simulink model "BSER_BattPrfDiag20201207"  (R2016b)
settings: Solver=FixedStepDiscrete  StartTime=0.0  StopTime=10.0  FixedStep=0.02  RelTol=1e-3  EnableMultiTasking=on
undefined symbols (not defined in the file or in its folder): bin2dec, BSER_cntBattOCMinDiag_C, BSER_cntBattPrfDiag_CW, BSER_cntChrgOCNpl_C, BSER_cntDisChOCNpl_C, BSER_cntPwrConvertConst_C, BSER_iChrgCurrErr_C, BSER_iChrgCurrOk_C, BSER_iDisChCurrErr_C, BSER_iDisChCurrOk_C, BSER_iLonChrgCurrErr_C, BSER_iLonChrgCurrOk_C, BSER_iLonDisChCurrErr_C, BSER_iLonDisChCurrOk_C, BSER_iShrtChrgCurrErr_C, BSER_iShrtChrgCurrOk_C, BSER_iShrtDisChCurrErr_C, BSER_iShrtDisChCurrOk_C, BSER_iSumLonChrgCurrReq_C, BSER_iSumLonDisChCurrReq_C, BSER_iSumShrtChrgCurrReq_C, BSER_iSumShrtDisChCurrReq_C, BSER_rLonChrgCurrHeal_C, BSER_rLonChrgCurrHi_C, BSER_rLonDisChCurrHeal_C, BSER_rLonDisChCurrHi_C, BSER_rShrtChrgCurrHeal_C, BSER_rShrtChrgCurrHi_C, BSER_rShrtDisChCurrHeal_C, BSER_rShrtDisChCurrHi_C, BSER_tiChrgCurrErr_C, BSER_tiChrgCurrOk_C, BSER_tiCurrConstPer_C, BSER_tiCurrPeakPer_C, BSER_tiDisChCurrErr_C, BSER_tiDisChCurrOk_C, BSER_uBattVoltConst_C
libraries: simulink x68
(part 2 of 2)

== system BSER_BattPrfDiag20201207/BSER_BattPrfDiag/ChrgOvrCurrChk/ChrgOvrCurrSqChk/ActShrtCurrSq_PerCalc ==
  BSPR_iCurr : Inport
  BSER_tiCurrConstPer_C : Inport  Port=2
  CurrProc : Stateflow chart  TreatAsAtomicUnit=on
  Sum of Elements : Sum  Inputs=+
  Terminator : Terminator
  Terminator1 : Terminator
  BSER_iCurrPerAcm : Outport
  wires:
  CurrProc/2(Index_s) -> Terminator/1
  CurrProc/3(i) -> Terminator1/1
  CurrProc/1(BSER_iCurrSqAvrgS_A) -> Sum of Elements/1
  BSPR_iCurr/1 -> CurrProc/1(BSPR_iCurr)
  Sum of Elements/1 -> BSER_iCurrPerAcm/1
  BSER_tiCurrConstPer_C/1 -> CurrProc/2(BSER_tiCurrCalcPer_C)

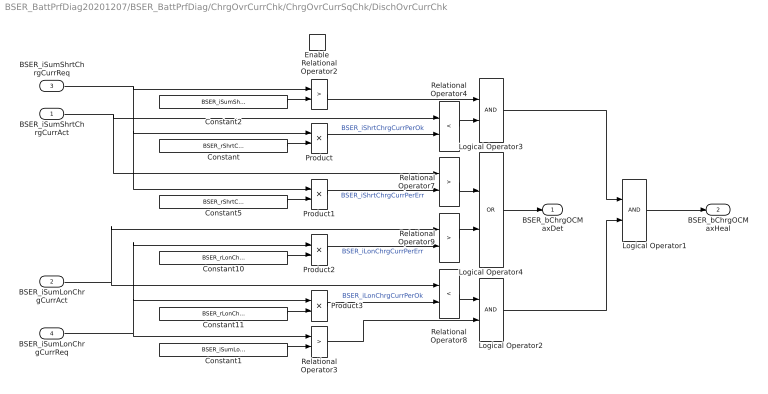
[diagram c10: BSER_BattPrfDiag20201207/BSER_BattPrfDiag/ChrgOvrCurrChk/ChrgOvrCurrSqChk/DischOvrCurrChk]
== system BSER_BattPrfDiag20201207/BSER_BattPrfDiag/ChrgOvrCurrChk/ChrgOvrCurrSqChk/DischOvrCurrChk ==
  BSER_iSumShrtChrgCurrAct : Inport
  BSER_iSumLonChrgCurrAct : Inport  Port=2
  BSER_iSumShrtChrgCurrReq : Inport  Port=3
  BSER_iSumLonChrgCurrReq : Inport  Port=4
  Enable : EnablePort
  Constant : Constant  Value=BSER_rShrtChrgCurrHeal_C
  Constant1 : Constant  Value=BSER_iSumLonChrgCurrReq_C
  Constant10 : Constant  Value=BSER_rLonChrgCurrHi_C
  Constant11 : Constant  Value=BSER_rLonChrgCurrHeal_C
  Constant2 : Constant  Value=BSER_iSumShrtChrgCurrReq_C
  Constant5 : Constant  Value=BSER_rShrtChrgCurrHi_C
  Logical Operator1 : Logic  AllPortsSameDT=off  OutDataTypeStr=boolean
  Logical Operator2 : Logic  AllPortsSameDT=off  OutDataTypeStr=boolean
  Logical Operator3 : Logic  AllPortsSameDT=off  OutDataTypeStr=boolean
  Logical Operator4 : Logic  Operator=OR  AllPortsSameDT=off  OutDataTypeStr=boolean
  Product{,1..3} (4 alike) : Product
  Relational Operator{2..3,7,9} (4 alike) : RelationalOperator  Operator=>  OutDataTypeStr=boolean  RndMeth=Simplest
  Relational Operator4 : RelationalOperator  Operator=<  OutDataTypeStr=boolean  RndMeth=Simplest
  Relational Operator8 : RelationalOperator  Operator=<  OutDataTypeStr=boolean  RndMeth=Simplest
  BSER_bChrgOCMaxDet : Outport
  BSER_bChrgOCMaxHeal : Outport  Port=2
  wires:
  Logical Operator1/1 -> BSER_bChrgOCMaxHeal/1
  Logical Operator4/1 -> BSER_bChrgOCMaxDet/1
  Logical Operator2/1 -> Logical Operator1/2
  Logical Operator3/1 -> Logical Operator1/1
  Relational Operator8/1 -> Logical Operator2/1
  Relational Operator3/1 -> Logical Operator2/2
  Relational Operator2/1 -> Logical Operator3/1
  Constant1/1 -> Relational Operator3/2
  Relational Operator4/1 -> Logical Operator3/2
  Relational Operator9/1 -> Logical Operator4/2
  Relational Operator7/1 -> Logical Operator4/1
  BSER_iSumLonChrgCurrAct/1 -> Relational Operator9/1, Relational Operator8/1
  BSER_iSumLonChrgCurrReq/1 -> Product3/1, Product2/1, Relational Operator3/1
  BSER_iSumShrtChrgCurrAct/1 -> Relational Operator7/1, Relational Operator4/1
  BSER_iSumShrtChrgCurrReq/1 -> Product1/1, Product/1, Relational Operator2/1
  Constant/1 -> Product/2
  Product/1 -> Relational Operator4/2  "BSER_iShrtChrgCurrPerOk"
  Product1/1 -> Relational Operator7/2  "BSER_iShrtChrgCurrPerErr"
  Constant5/1 -> Product1/2
  Constant2/1 -> Relational Operator2/2
  Constant10/1 -> Product2/2
  Product2/1 -> Relational Operator9/2  "BSER_iLonChrgCurrPerErr"
  Product3/1 -> Relational Operator8/2  "BSER_iLonChrgCurrPerOk"
  Constant11/1 -> Product3/2

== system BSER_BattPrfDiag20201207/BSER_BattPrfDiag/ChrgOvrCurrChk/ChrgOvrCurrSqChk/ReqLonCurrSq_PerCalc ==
  BSPR_iCurr : Inport
  BSER_tiCurrConstPer_C : Inport  Port=2
  CurrProc1 : Stateflow chart  TreatAsAtomicUnit=on
  Sum of Elements : Sum  Inputs=+
  Terminator : Terminator
  Terminator1 : Terminator
  BSER_iCurrPerAcm : Outport
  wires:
  BSER_tiCurrConstPer_C/1 -> CurrProc1/2(BSER_tiCurrCalcPer_C)
  Sum of Elements/1 -> BSER_iCurrPerAcm/1
  BSPR_iCurr/1 -> CurrProc1/1(BSPR_iCurr)
  CurrProc1/1(BSER_iCurrSqAvrgS_A) -> Sum of Elements/1
  CurrProc1/3(i) -> Terminator1/1
  CurrProc1/2(Index_s) -> Terminator/1

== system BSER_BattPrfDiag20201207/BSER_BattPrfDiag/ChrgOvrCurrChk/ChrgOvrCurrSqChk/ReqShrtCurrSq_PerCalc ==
  BSPR_iCurr : Inport
  BSER_tiCurrConstPer_C : Inport  Port=2
  CurrProc : Stateflow chart  TreatAsAtomicUnit=on
  Sum of Elements : Sum  Inputs=+
  Terminator : Terminator
  Terminator1 : Terminator
  BSER_iCurrPerAcm : Outport
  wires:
  CurrProc/2(Index_s) -> Terminator/1
  CurrProc/3(i) -> Terminator1/1
  CurrProc/1(BSER_iCurrSqAvrgS_A) -> Sum of Elements/1
  BSPR_iCurr/1 -> CurrProc/1(BSPR_iCurr)
  Sum of Elements/1 -> BSER_iCurrPerAcm/1
  BSER_tiCurrConstPer_C/1 -> CurrProc/2(BSER_tiCurrCalcPer_C)

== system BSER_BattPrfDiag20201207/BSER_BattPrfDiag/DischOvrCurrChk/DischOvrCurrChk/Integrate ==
  In : Inport
  Add : Sum
  Delay : Delay  DelayLength=1  InitialCondition=0
  Gain : Gain  Gain=0.01
  Saturation : Saturate  UpperLimit=50000  LowerLimit=0
  Out : Outport
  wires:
  Saturation/1 -> Delay/1, Out/1
  In/1 -> Gain/1
  Delay/1 -> Add/1
  Add/1 -> Saturation/1
  Gain/1 -> Add/2

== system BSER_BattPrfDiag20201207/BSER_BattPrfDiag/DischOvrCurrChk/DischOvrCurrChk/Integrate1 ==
  In : Inport
  Add : Sum
  Delay : Delay  DelayLength=1  InitialCondition=0
  Gain : Gain  Gain=0.01
  Saturation : Saturate  UpperLimit=25000  LowerLimit=0
  Out : Outport
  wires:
  Add/1 -> Saturation/1
  Delay/1 -> Add/1
  In/1 -> Gain/1
  Saturation/1 -> Out/1, Delay/1
  Gain/1 -> Add/2

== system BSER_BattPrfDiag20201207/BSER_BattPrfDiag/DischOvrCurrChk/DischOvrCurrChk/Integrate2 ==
  In : Inport
  Add : Sum
  Delay : Delay  DelayLength=1  InitialCondition=0
  Gain : Gain  Gain=0.01
  Saturation : Saturate  UpperLimit=50000  LowerLimit=0
  Out : Outport
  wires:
  Saturation/1 -> Delay/1, Out/1
  In/1 -> Gain/1
  Delay/1 -> Add/1
  Add/1 -> Saturation/1
  Gain/1 -> Add/2

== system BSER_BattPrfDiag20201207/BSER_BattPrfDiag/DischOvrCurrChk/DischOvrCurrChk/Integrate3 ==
  In : Inport
  Add : Sum
  Delay : Delay  DelayLength=1  InitialCondition=0
  Gain : Gain  Gain=0.01
  Saturation : Saturate  UpperLimit=25000  LowerLimit=0
  Out : Outport
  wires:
  Add/1 -> Saturation/1
  Delay/1 -> Add/1
  In/1 -> Gain/1
  Saturation/1 -> Out/1, Delay/1
  Gain/1 -> Add/2

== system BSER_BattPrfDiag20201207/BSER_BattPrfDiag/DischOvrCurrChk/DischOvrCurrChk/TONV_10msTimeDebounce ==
  note: Turn On Delay Time Deboune
  u : Inport
  T : Inport  Port=2
  Add : Sum
  Constant1 : Constant  Value=0  OutDataTypeStr=single
  Constant2 : Constant  OutDataTypeStr=uint8
  Constant3 : Constant  Value=0  OutDataTypeStr=uint8
  Constant4 : Constant  Value=0.01  OutDataTypeStr=single
  Delay : Delay  DelayLength=1  InitialCondition=0
  MinMax : MinMax  Inputs=2
  Product : Product  OutMin=[0]  OutMax=[65535]  OutDataTypeStr=single
  Relational Operator : RelationalOperator  Operator=>  OutDataTypeStr=boolean  RndMeth=Simplest
  Switch : Switch  Criteria=u2 ~= 0
  Switch1 : Switch  Criteria=u2 ~= 0
  y : Outport
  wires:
  MinMax/1 -> Add/2
  T/1 -> Relational Operator/2, MinMax/1
  Relational Operator/1 -> y/1
  Delay/1 -> MinMax/2
  Switch/1 -> Add/1
  Product/1 -> Delay/1, Relational Operator/1
  Add/1 -> Product/2
  Constant1/1 -> Switch/3
  Constant4/1 -> Switch/1
  u/1 -> Switch/2, Switch1/2
  Constant2/1 -> Switch1/1
  Constant3/1 -> Switch1/3
  Switch1/1 -> Product/1

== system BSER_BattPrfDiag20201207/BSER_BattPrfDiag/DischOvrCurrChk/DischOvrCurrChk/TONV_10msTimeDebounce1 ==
  note: Turn On Delay Time Deboune
  u : Inport
  T : Inport  Port=2
  Add : Sum
  Constant1 : Constant  Value=0  OutDataTypeStr=single
  Constant2 : Constant  OutDataTypeStr=uint8
  Constant3 : Constant  Value=0  OutDataTypeStr=uint8
  Constant4 : Constant  Value=0.01  OutDataTypeStr=single
  Delay : Delay  DelayLength=1  InitialCondition=0
  MinMax : MinMax  Inputs=2
  Product : Product  OutMin=[0]  OutMax=[65535]  OutDataTypeStr=single
  Relational Operator : RelationalOperator  Operator=>  OutDataTypeStr=boolean  RndMeth=Simplest
  Switch : Switch  Criteria=u2 ~= 0
  Switch1 : Switch  Criteria=u2 ~= 0
  y : Outport
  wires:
  Switch1/1 -> Product/1
  Constant3/1 -> Switch1/3
  Constant2/1 -> Switch1/1
  u/1 -> Switch1/2, Switch/2
  Constant4/1 -> Switch/1
  Constant1/1 -> Switch/3
  Add/1 -> Product/2
  Product/1 -> Relational Operator/1, Delay/1
  Switch/1 -> Add/1
  Delay/1 -> MinMax/2
  Relational Operator/1 -> y/1
  T/1 -> MinMax/1, Relational Operator/2
  MinMax/1 -> Add/2

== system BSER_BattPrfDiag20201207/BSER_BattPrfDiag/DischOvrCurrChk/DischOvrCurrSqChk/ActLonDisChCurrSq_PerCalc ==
  BSPR_iCurr : Inport
  BSER_tiCurrConstPer_C : Inport  Port=2
  CurrProc : Stateflow chart  TreatAsAtomicUnit=on
  Sum of Elements : Sum  Inputs=+
  Terminator : Terminator
  Terminator1 : Terminator
  BSER_iCurrPerAcm : Outport
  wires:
  BSER_tiCurrConstPer_C/1 -> CurrProc/2(BSER_tiCurrCalcPer_C)
  Sum of Elements/1 -> BSER_iCurrPerAcm/1
  BSPR_iCurr/1 -> CurrProc/1(BSPR_iCurr)
  CurrProc/1(BSER_iCurrSqAvrgS_A) -> Sum of Elements/1
  CurrProc/3(i) -> Terminator1/1
  CurrProc/2(Index_s) -> Terminator/1

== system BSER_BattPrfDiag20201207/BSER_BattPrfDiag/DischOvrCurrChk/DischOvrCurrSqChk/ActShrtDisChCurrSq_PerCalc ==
  BSPR_iCurr : Inport
  BSER_tiCurrConstPer_C : Inport  Port=2
  CurrProc : Stateflow chart  TreatAsAtomicUnit=on
  Sum of Elements : Sum  Inputs=+
  Terminator : Terminator
  Terminator1 : Terminator
  BSER_iCurrPerAcm : Outport
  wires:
  CurrProc/2(Index_s) -> Terminator/1
  CurrProc/3(i) -> Terminator1/1
  CurrProc/1(BSER_iCurrSqAvrgS_A) -> Sum of Elements/1
  BSPR_iCurr/1 -> CurrProc/1(BSPR_iCurr)
  Sum of Elements/1 -> BSER_iCurrPerAcm/1
  BSER_tiCurrConstPer_C/1 -> CurrProc/2(BSER_tiCurrCalcPer_C)

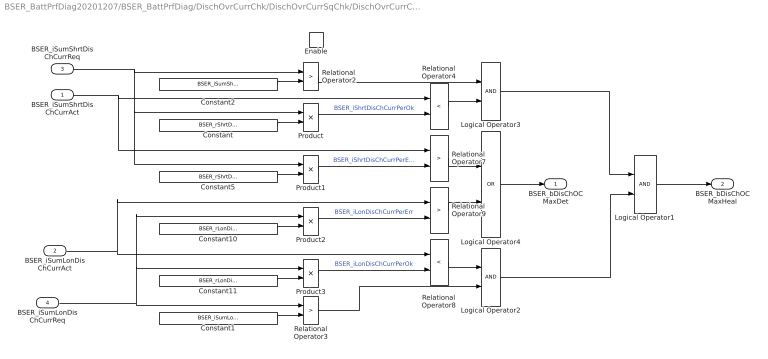
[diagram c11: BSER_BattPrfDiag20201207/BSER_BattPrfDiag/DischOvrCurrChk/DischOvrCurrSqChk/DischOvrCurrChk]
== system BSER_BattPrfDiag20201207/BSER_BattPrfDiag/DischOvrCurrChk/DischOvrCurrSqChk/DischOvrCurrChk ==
  BSER_iSumShrtDisChCurrAct : Inport
  BSER_iSumLonDisChCurrAct : Inport  Port=2
  BSER_iSumShrtDisChCurrReq : Inport  Port=3
  BSER_iSumLonDisChCurrReq : Inport  Port=4
  Enable : EnablePort
  Constant : Constant  Value=BSER_rShrtDisChCurrHeal_C
  Constant1 : Constant  Value=BSER_iSumLonDisChCurrReq_C
  Constant10 : Constant  Value=BSER_rLonDisChCurrHi_C
  Constant11 : Constant  Value=BSER_rLonDisChCurrHeal_C
  Constant2 : Constant  Value=BSER_iSumShrtDisChCurrReq_C
  Constant5 : Constant  Value=BSER_rShrtDisChCurrHi_C
  Logical Operator1 : Logic  AllPortsSameDT=off  OutDataTypeStr=boolean
  Logical Operator2 : Logic  AllPortsSameDT=off  OutDataTypeStr=boolean
  Logical Operator3 : Logic  AllPortsSameDT=off  OutDataTypeStr=boolean
  Logical Operator4 : Logic  Operator=OR  AllPortsSameDT=off  OutDataTypeStr=boolean
  Product{,1..3} (4 alike) : Product
  Relational Operator{2..3,7,9} (4 alike) : RelationalOperator  Operator=>  OutDataTypeStr=boolean  RndMeth=Simplest
  Relational Operator4 : RelationalOperator  Operator=<  OutDataTypeStr=boolean  RndMeth=Simplest
  Relational Operator8 : RelationalOperator  Operator=<  OutDataTypeStr=boolean  RndMeth=Simplest
  BSER_bDisChOCMaxDet : Outport
  BSER_bDisChOCMaxHeal : Outport  Port=2
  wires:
  BSER_iSumShrtDisChCurrAct/1 -> Relational Operator4/1, Relational Operator7/1
  BSER_iSumShrtDisChCurrReq/1 -> Relational Operator2/1, Product/1, Product1/1
  BSER_iSumLonDisChCurrAct/1 -> Relational Operator8/1, Relational Operator9/1
  BSER_iSumLonDisChCurrReq/1 -> Relational Operator3/1, Product3/1, Product2/1
  Relational Operator7/1 -> Logical Operator4/1
  Relational Operator9/1 -> Logical Operator4/2
  Relational Operator4/1 -> Logical Operator3/2
  Constant1/1 -> Relational Operator3/2
  Relational Operator2/1 -> Logical Operator3/1
  Relational Operator3/1 -> Logical Operator2/2
  Relational Operator8/1 -> Logical Operator2/1
  Logical Operator3/1 -> Logical Operator1/1
  Logical Operator2/1 -> Logical Operator1/2
  Logical Operator4/1 -> BSER_bDisChOCMaxDet/1
  Logical Operator1/1 -> BSER_bDisChOCMaxHeal/1
  Constant2/1 -> Relational Operator2/2
  Constant/1 -> Product/2
  Product/1 -> Relational Operator4/2  "BSER_iShrtDisChCurrPerOk"
  Product1/1 -> Relational Operator7/2  "BSER_iShrtDisChCurrPerErr"
  Constant5/1 -> Product1/2
  Constant10/1 -> Product2/2
  Product2/1 -> Relational Operator9/2  "BSER_iLonDisChCurrPerErr"
  Product3/1 -> Relational Operator8/2  "BSER_iLonDisChCurrPerOk"
  Constant11/1 -> Product3/2

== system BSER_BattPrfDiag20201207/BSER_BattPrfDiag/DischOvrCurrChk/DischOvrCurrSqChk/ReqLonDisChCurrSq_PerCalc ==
  BSPR_iCurr : Inport
  BSER_tiCurrConstPer_C : Inport  Port=2
  CurrProc : Stateflow chart  TreatAsAtomicUnit=on
  Sum of Elements : Sum  Inputs=+
  Terminator : Terminator
  Terminator1 : Terminator
  BSER_iCurrPerAcm : Outport
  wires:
  BSER_tiCurrConstPer_C/1 -> CurrProc/2(BSER_tiCurrCalcPer_C)
  Sum of Elements/1 -> BSER_iCurrPerAcm/1
  BSPR_iCurr/1 -> CurrProc/1(BSPR_iCurr)
  CurrProc/1(BSER_iCurrSqAvrgS_A) -> Sum of Elements/1
  CurrProc/3(i) -> Terminator1/1
  CurrProc/2(Index_s) -> Terminator/1

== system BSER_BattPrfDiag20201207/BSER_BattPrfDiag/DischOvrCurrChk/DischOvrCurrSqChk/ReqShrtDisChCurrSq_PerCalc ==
  BSPR_iCurr : Inport
  BSER_tiCurrConstPer_C : Inport  Port=2
  CurrProc : Stateflow chart  TreatAsAtomicUnit=on
  Sum of Elements : Sum  Inputs=+
  Terminator : Terminator
  Terminator1 : Terminator
  BSER_iCurrPerAcm : Outport
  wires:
  CurrProc/2(Index_s) -> Terminator/1
  CurrProc/3(i) -> Terminator1/1
  CurrProc/1(BSER_iCurrSqAvrgS_A) -> Sum of Elements/1
  BSPR_iCurr/1 -> CurrProc/1(BSPR_iCurr)
  Sum of Elements/1 -> BSER_iCurrPerAcm/1
  BSER_tiCurrConstPer_C/1 -> CurrProc/2(BSER_tiCurrCalcPer_C)

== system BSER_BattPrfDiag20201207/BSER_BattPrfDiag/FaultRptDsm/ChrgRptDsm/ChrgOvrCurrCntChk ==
  BSER_bChrgOCMaxDet : Inport
  BSER_bChrgOCMinDet : Inport  Port=2
  Constant3 : Constant  Value=0  OutDataTypeStr=uint8
  Constant4 : Constant  OutDataTypeStr=uint8
  Constant5 : Constant  Value=BSER_cntChrgOCNpl_C
  Delay : Delay  DelayLength=1  InitialCondition=0
  EdgeRising : Subsystem  TreatAsAtomicUnit=on  RTWFcnName=EdgeRising  RTWFileName=SrvLib
  Logical Operator3 : Logic  Operator=NOT  AllPortsSameDT=off  OutDataTypeStr=boolean
  Logical Operator4 : Logic  Operator=OR  AllPortsSameDT=off  OutDataTypeStr=boolean
  Relational Operator7 : RelationalOperator  Operator=>  OutDataTypeStr=boolean  RndMeth=Simplest
  Subtract : Sum  OutDataTypeStr=uint8
  Switch : Switch  Criteria=u2 > Threshold
  BSER_bChrgOCNplHeal : Outport
  BSER_bChrgOCNplDet : Outport  Port=2
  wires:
  Relational Operator7/1 -> BSER_bChrgOCNplDet/1, Logical Operator3/1
  Delay/1 -> Subtract/2
  Subtract/1 -> Delay/1, Relational Operator7/1  "BSER_cntChrgOCNpl"
  Switch/1 -> Subtract/1
  EdgeRising/1(y) -> Switch/2
  Constant4/1 -> Switch/1
  Constant3/1 -> Switch/3
  Constant5/1 -> Relational Operator7/2
  Logical Operator3/1 -> BSER_bChrgOCNplHeal/1
  Logical Operator4/1 -> EdgeRising/1(u)
  BSER_bChrgOCMaxDet/1 -> Logical Operator4/1
  BSER_bChrgOCMinDet/1 -> Logical Operator4/2

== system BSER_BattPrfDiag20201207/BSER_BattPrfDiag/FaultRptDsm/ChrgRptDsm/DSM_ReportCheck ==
  note: Fault report to diagnostic management system
  Dfc_id_nv : Inport  OutDataTypeStr=uint8
  Err : Inport  Port=2
  Heal : Inport  Port=3
  Bit Clear1 : simulink/Logic and Bit Operations/Bit Clear  iBit=4
  Bit Clear2 : simulink/Logic and Bit Operations/Bit Clear  iBit=3
  Bit Set : simulink/Logic and Bit Operations/Bit Set  iBit=4
  Bit Set1 : simulink/Logic and Bit Operations/Bit Set  iBit=3
  Bit Set2 : simulink/Logic and Bit Operations/Bit Set  iBit=3
  Bit Set4 : simulink/Logic and Bit Operations/Bit Set  iBit=7
  Constant7 : Constant  Value=0  OutDataTypeStr=boolean
  Delay2 : Delay  DelayLength=1  InitialCondition=1
  Delay3 : Delay  DelayLength=1  InitialCondition=0
  Switch2 : Switch  Criteria=u2 ~= 0
  Switch3 : Switch  Criteria=u2 ~= 0
  Switch4 : Switch  Criteria=u2 ~= 0
  Dfc_id : Outport  OutDataTypeStr=uint8
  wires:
  Dfc_id_nv/1 -> Bit Clear2/1, Bit Set4/1, Bit Clear1/1
  Bit Set4/1 -> Bit Set/1
  Constant7/1 -> Delay2/1
  Delay2/1 -> Switch2/2
  Switch3/1 -> Switch2/3
  Bit Clear2/1 -> Switch2/1
  Switch2/1 -> Delay3/1, Dfc_id/1
  Bit Set1/1 -> Switch3/1
  Bit Set/1 -> Bit Set1/1
  Switch4/1 -> Switch3/3
  Err/1 -> Switch3/2
  Bit Set2/1 -> Switch4/1
  Bit Clear1/1 -> Bit Set2/1
  Delay3/1 -> Switch4/3
  Heal/1 -> Switch4/2

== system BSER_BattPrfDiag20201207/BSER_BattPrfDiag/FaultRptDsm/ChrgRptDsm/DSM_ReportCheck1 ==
  note: Fault report to diagnostic management system
  Dfc_id_nv : Inport  OutDataTypeStr=uint8
  Err : Inport  Port=2
  Heal : Inport  Port=3
  Bit Clear1 : simulink/Logic and Bit Operations/Bit Clear  iBit=4
  Bit Clear2 : simulink/Logic and Bit Operations/Bit Clear  iBit=3
  Bit Set : simulink/Logic and Bit Operations/Bit Set  iBit=4
  Bit Set1 : simulink/Logic and Bit Operations/Bit Set  iBit=3
  Bit Set2 : simulink/Logic and Bit Operations/Bit Set  iBit=3
  Bit Set4 : simulink/Logic and Bit Operations/Bit Set  iBit=7
  Constant7 : Constant  Value=0  OutDataTypeStr=boolean
  Delay2 : Delay  DelayLength=1  InitialCondition=1
  Delay3 : Delay  DelayLength=1  InitialCondition=0
  Switch2 : Switch  Criteria=u2 ~= 0
  Switch3 : Switch  Criteria=u2 ~= 0
  Switch4 : Switch  Criteria=u2 ~= 0
  Dfc_id : Outport  OutDataTypeStr=uint8
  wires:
  Heal/1 -> Switch4/2
  Delay3/1 -> Switch4/3
  Bit Clear1/1 -> Bit Set2/1
  Bit Set2/1 -> Switch4/1
  Err/1 -> Switch3/2
  Switch4/1 -> Switch3/3
  Bit Set/1 -> Bit Set1/1
  Bit Set1/1 -> Switch3/1
  Switch2/1 -> Dfc_id/1, Delay3/1
  Bit Clear2/1 -> Switch2/1
  Switch3/1 -> Switch2/3
  Delay2/1 -> Switch2/2
  Constant7/1 -> Delay2/1
  Bit Set4/1 -> Bit Set/1
  Dfc_id_nv/1 -> Bit Clear1/1, Bit Set4/1, Bit Clear2/1

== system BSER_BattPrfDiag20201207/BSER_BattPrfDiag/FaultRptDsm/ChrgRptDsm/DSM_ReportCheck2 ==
  note: Fault report to diagnostic management system
  Dfc_id_nv : Inport  OutDataTypeStr=uint8
  Err : Inport  Port=2
  Heal : Inport  Port=3
  Bit Clear1 : simulink/Logic and Bit Operations/Bit Clear  iBit=4
  Bit Clear2 : simulink/Logic and Bit Operations/Bit Clear  iBit=3
  Bit Set : simulink/Logic and Bit Operations/Bit Set  iBit=4
  Bit Set1 : simulink/Logic and Bit Operations/Bit Set  iBit=3
  Bit Set2 : simulink/Logic and Bit Operations/Bit Set  iBit=3
  Bit Set4 : simulink/Logic and Bit Operations/Bit Set  iBit=7
  Constant7 : Constant  Value=0  OutDataTypeStr=boolean
  Delay2 : Delay  DelayLength=1  InitialCondition=1
  Delay3 : Delay  DelayLength=1  InitialCondition=0
  Switch2 : Switch  Criteria=u2 ~= 0
  Switch3 : Switch  Criteria=u2 ~= 0
  Switch4 : Switch  Criteria=u2 ~= 0
  Dfc_id : Outport  OutDataTypeStr=uint8
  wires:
  Dfc_id_nv/1 -> Bit Clear2/1, Bit Set4/1, Bit Clear1/1
  Bit Set4/1 -> Bit Set/1
  Constant7/1 -> Delay2/1
  Delay2/1 -> Switch2/2
  Switch3/1 -> Switch2/3
  Bit Clear2/1 -> Switch2/1
  Switch2/1 -> Delay3/1, Dfc_id/1
  Bit Set1/1 -> Switch3/1
  Bit Set/1 -> Bit Set1/1
  Switch4/1 -> Switch3/3
  Err/1 -> Switch3/2
  Bit Set2/1 -> Switch4/1
  Bit Clear1/1 -> Bit Set2/1
  Delay3/1 -> Switch4/3
  Heal/1 -> Switch4/2

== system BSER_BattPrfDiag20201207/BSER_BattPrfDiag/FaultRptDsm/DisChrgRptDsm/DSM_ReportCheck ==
  note: Fault report to diagnostic management system
  Dfc_id_nv : Inport  OutDataTypeStr=uint8
  Err : Inport  Port=2
  Heal : Inport  Port=3
  Bit Clear1 : simulink/Logic and Bit Operations/Bit Clear  iBit=4
  Bit Clear2 : simulink/Logic and Bit Operations/Bit Clear  iBit=3
  Bit Set : simulink/Logic and Bit Operations/Bit Set  iBit=4
  Bit Set1 : simulink/Logic and Bit Operations/Bit Set  iBit=3
  Bit Set2 : simulink/Logic and Bit Operations/Bit Set  iBit=3
  Bit Set4 : simulink/Logic and Bit Operations/Bit Set  iBit=7
  Constant7 : Constant  Value=0  OutDataTypeStr=boolean
  Delay2 : Delay  DelayLength=1  InitialCondition=1
  Delay3 : Delay  DelayLength=1  InitialCondition=0
  Switch2 : Switch  Criteria=u2 ~= 0
  Switch3 : Switch  Criteria=u2 ~= 0
  Switch4 : Switch  Criteria=u2 ~= 0
  Dfc_id : Outport  OutDataTypeStr=uint8
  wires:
  Dfc_id_nv/1 -> Bit Clear2/1, Bit Set4/1, Bit Clear1/1
  Bit Set4/1 -> Bit Set/1
  Constant7/1 -> Delay2/1
  Delay2/1 -> Switch2/2
  Switch3/1 -> Switch2/3
  Bit Clear2/1 -> Switch2/1
  Switch2/1 -> Delay3/1, Dfc_id/1
  Bit Set1/1 -> Switch3/1
  Bit Set/1 -> Bit Set1/1
  Switch4/1 -> Switch3/3
  Err/1 -> Switch3/2
  Bit Set2/1 -> Switch4/1
  Bit Clear1/1 -> Bit Set2/1
  Delay3/1 -> Switch4/3
  Heal/1 -> Switch4/2

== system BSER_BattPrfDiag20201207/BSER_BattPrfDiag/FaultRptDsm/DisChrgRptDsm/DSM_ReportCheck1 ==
  note: Fault report to diagnostic management system
  Dfc_id_nv : Inport  OutDataTypeStr=uint8
  Err : Inport  Port=2
  Heal : Inport  Port=3
  Bit Clear1 : simulink/Logic and Bit Operations/Bit Clear  iBit=4
  Bit Clear2 : simulink/Logic and Bit Operations/Bit Clear  iBit=3
  Bit Set : simulink/Logic and Bit Operations/Bit Set  iBit=4
  Bit Set1 : simulink/Logic and Bit Operations/Bit Set  iBit=3
  Bit Set2 : simulink/Logic and Bit Operations/Bit Set  iBit=3
  Bit Set4 : simulink/Logic and Bit Operations/Bit Set  iBit=7
  Constant7 : Constant  Value=0  OutDataTypeStr=boolean
  Delay2 : Delay  DelayLength=1  InitialCondition=1
  Delay3 : Delay  DelayLength=1  InitialCondition=0
  Switch2 : Switch  Criteria=u2 ~= 0
  Switch3 : Switch  Criteria=u2 ~= 0
  Switch4 : Switch  Criteria=u2 ~= 0
  Dfc_id : Outport  OutDataTypeStr=uint8
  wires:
  Heal/1 -> Switch4/2
  Delay3/1 -> Switch4/3
  Bit Clear1/1 -> Bit Set2/1
  Bit Set2/1 -> Switch4/1
  Err/1 -> Switch3/2
  Switch4/1 -> Switch3/3
  Bit Set/1 -> Bit Set1/1
  Bit Set1/1 -> Switch3/1
  Switch2/1 -> Dfc_id/1, Delay3/1
  Bit Clear2/1 -> Switch2/1
  Switch3/1 -> Switch2/3
  Delay2/1 -> Switch2/2
  Constant7/1 -> Delay2/1
  Bit Set4/1 -> Bit Set/1
  Dfc_id_nv/1 -> Bit Clear1/1, Bit Set4/1, Bit Clear2/1

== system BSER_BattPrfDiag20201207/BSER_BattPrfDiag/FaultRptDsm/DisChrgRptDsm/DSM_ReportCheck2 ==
  note: Fault report to diagnostic management system
  Dfc_id_nv : Inport  OutDataTypeStr=uint8
  Err : Inport  Port=2
  Heal : Inport  Port=3
  Bit Clear1 : simulink/Logic and Bit Operations/Bit Clear  iBit=4
  Bit Clear2 : simulink/Logic and Bit Operations/Bit Clear  iBit=3
  Bit Set : simulink/Logic and Bit Operations/Bit Set  iBit=4
  Bit Set1 : simulink/Logic and Bit Operations/Bit Set  iBit=3
  Bit Set2 : simulink/Logic and Bit Operations/Bit Set  iBit=3
  Bit Set4 : simulink/Logic and Bit Operations/Bit Set  iBit=7
  Constant7 : Constant  Value=0  OutDataTypeStr=boolean
  Delay2 : Delay  DelayLength=1  InitialCondition=1
  Delay3 : Delay  DelayLength=1  InitialCondition=0
  Switch2 : Switch  Criteria=u2 ~= 0
  Switch3 : Switch  Criteria=u2 ~= 0
  Switch4 : Switch  Criteria=u2 ~= 0
  Dfc_id : Outport  OutDataTypeStr=uint8
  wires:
  Dfc_id_nv/1 -> Bit Clear2/1, Bit Set4/1, Bit Clear1/1
  Bit Set4/1 -> Bit Set/1
  Constant7/1 -> Delay2/1
  Delay2/1 -> Switch2/2
  Switch3/1 -> Switch2/3
  Bit Clear2/1 -> Switch2/1
  Switch2/1 -> Delay3/1, Dfc_id/1
  Bit Set1/1 -> Switch3/1
  Bit Set/1 -> Bit Set1/1
  Switch4/1 -> Switch3/3
  Err/1 -> Switch3/2
  Bit Set2/1 -> Switch4/1
  Bit Clear1/1 -> Bit Set2/1
  Delay3/1 -> Switch4/3
  Heal/1 -> Switch4/2

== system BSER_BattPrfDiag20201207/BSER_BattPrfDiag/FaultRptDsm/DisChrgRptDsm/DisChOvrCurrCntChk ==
  BSER_bDisChOCMaxDet : Inport
  BSER_bDisChOCMinDet : Inport  Port=2
  Constant3 : Constant  Value=0  OutDataTypeStr=uint8
  Constant4 : Constant  OutDataTypeStr=uint8
  Constant5 : Constant  Value=BSER_cntDisChOCNpl_C
  Delay : Delay  DelayLength=1  InitialCondition=0
  EdgeRising : Subsystem  TreatAsAtomicUnit=on  RTWFcnName=EdgeRising  RTWFileName=SrvLib
  Logical Operator3 : Logic  Operator=NOT  AllPortsSameDT=off  OutDataTypeStr=boolean
  Logical Operator4 : Logic  Operator=OR  AllPortsSameDT=off  OutDataTypeStr=boolean
  Relational Operator7 : RelationalOperator  OutDataTypeStr=boolean  RndMeth=Simplest
  Subtract : Sum  OutDataTypeStr=uint8
  Switch : Switch  Criteria=u2 > Threshold
  BSER_bDisChOCNplHeal : Outport
  BSER_bDisChOCNplDet : Outport  Port=2
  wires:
  Logical Operator3/1 -> BSER_bDisChOCNplHeal/1
  Constant5/1 -> Relational Operator7/2
  Constant3/1 -> Switch/3
  Constant4/1 -> Switch/1
  EdgeRising/1(y) -> Switch/2
  Switch/1 -> Subtract/1
  Subtract/1 -> Delay/1, Relational Operator7/1  "BSER_cntDisChOCNpl"
  Delay/1 -> Subtract/2
  Relational Operator7/1 -> BSER_bDisChOCNplDet/1, Logical Operator3/1
  Logical Operator4/1 -> EdgeRising/1(u)
  BSER_bDisChOCMaxDet/1 -> Logical Operator4/1
  BSER_bDisChOCMinDet/1 -> Logical Operator4/2

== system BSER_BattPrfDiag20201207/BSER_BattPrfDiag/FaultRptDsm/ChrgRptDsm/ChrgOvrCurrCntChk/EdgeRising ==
  u : Inport
  Delay1 : Delay  DelayLength=1  InitialCondition=1
  Logical Operator3 : Logic  Operator=NOT  AllPortsSameDT=off  OutDataTypeStr=boolean
  Logical Operator4 : Logic  AllPortsSameDT=off  OutDataTypeStr=boolean
  y : Outport
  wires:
  Logical Operator4/1 -> y/1
  Logical Operator3/1 -> Logical Operator4/1
  u/1 -> Delay1/1, Logical Operator4/2
  Delay1/1 -> Logical Operator3/1

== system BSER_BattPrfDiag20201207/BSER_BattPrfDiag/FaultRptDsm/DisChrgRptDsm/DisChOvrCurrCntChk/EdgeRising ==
  u : Inport
  Delay1 : Delay  DelayLength=1  InitialCondition=1
  Logical Operator3 : Logic  Operator=NOT  AllPortsSameDT=off  OutDataTypeStr=boolean
  Logical Operator4 : Logic  AllPortsSameDT=off  OutDataTypeStr=boolean
  y : Outport
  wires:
  Logical Operator4/1 -> y/1
  Logical Operator3/1 -> Logical Operator4/1
  u/1 -> Delay1/1, Logical Operator4/2
  Delay1/1 -> Logical Operator3/1

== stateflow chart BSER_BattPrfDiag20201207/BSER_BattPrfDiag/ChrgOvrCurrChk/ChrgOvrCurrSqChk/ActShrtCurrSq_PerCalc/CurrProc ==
  state Time10msStrt_stt1
    entry:
    BSER_iCurrSqProcTmp=BSPR_iCurr*BSPR_iCurr;
    BSER_cntCurrSqProc=0;
  state Time100msProc_stt
    entry:
    BSER_iCurrSqProcTmp_A[i]=BSER_iCurrSqProcTmp/10;
    BSER_iCurrSqProcTmp=BSPR_iCurr*BSPR_iCurr;
    BSER_cntCurrSqProc=0;
  state Time10msProc_stt
    entry:
    BSER_iCurrSqProcTmp=BSER_iCurrSqProcTmp+BSPR_iCurr*BSPR_iCurr;
    BSER_cntCurrSqProc=BSER_cntCurrSqProc+1;
    during:
    BSER_iCurrSqProcTmp=BSER_iCurrSqProcTmp+BSPR_iCurr*BSPR_iCurr;
    BSER_cntCurrSqProc=BSER_cntCurrSqProc+1;
  (default) -> (junction 67) : {i=0;}
  (junction 67) -> (junction 70) : [i<=9]
  (junction 70) -> (junction 71) : {BSER_iCurrSqProcTmp_A[i]=0;}
  (junction 71) -> (junction 67) : {i = i + 1;}
  (junction 67) -> (junction 68) : {Index_s=0;}
  (junction 68) -> (junction 78) : [Index_s<60]
  (junction 78) -> (junction 77) : {BSER_iCurrSqAvrgS_A[Index_s]=0;}
  (junction 77) -> (junction 68) : {Index_s = Index_s + 1;}
  (junction 68) -> Time10msStrt_stt1 : {i=0; Index_s=0;}
  Time10msStrt_stt1 -> Time10msProc_stt
  Time10msProc_stt -> Time100msProc_stt : [BSER_cntCurrSqProc>=9]
  (junction 43) -> Time10msProc_stt
  Time100msProc_stt -> (junction 43) : {i=i+1;}
  (junction 43) -> (junction 41) : [i>9]
  (junction 52) -> Time10msProc_stt : {Index_s=0;}
  (junction 55) -> Time10msProc_stt
  (junction 41) -> (junction 83) : {i=0;BSER_iCurrSqAvrgS=0;}
  (junction 36) -> (junction 83) : {i = i + 1;}
  (junction 83) -> (junction 38)
  (junction 39) -> (junction 36) : {BSER_iCurrSqAvrgS=BSER_iCurrSqAvrgS... +BSER_iCurrSqProcTmp_A[i];}
  (junction 55) -> (junction 52) : [Index_s>=BSER_tiCurrCalcPer_C]
  (junction 38) -> (junction 55) : {i=0; BSER_iCurrSqAvrgS_A[Index_s]=BSER_iCurrSqAvrgS/10; Index_s=Index_s+1;}
  (junction 38) -> (junction 39) : [i<=9]
  data: BSER_iCurrSqProcTmp_A local single; BSER_iCurrSqAvrgS local single; BSER_iCurrSqAvrgS_A output single; Index_s output uint8; BSPR_iCurr input; BSER_tiCurrCalcPer_C input; BSER_iCurrSqProcTmp local single; i output uint8; BSER_cntCurrSqProc local uint8

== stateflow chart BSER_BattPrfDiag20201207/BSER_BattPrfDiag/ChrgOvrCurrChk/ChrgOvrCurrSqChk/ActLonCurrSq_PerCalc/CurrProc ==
  state Time10msStrt_stt1
    entry:
    BSER_iCurrSqProcTmp=BSPR_iCurr*BSPR_iCurr;
    BSER_cntCurrSqProc=0;
  state Time100msProc_stt
    entry:
    BSER_iCurrSqProcTmp_A[i]=BSER_iCurrSqProcTmp/10;
    BSER_iCurrSqProcTmp=BSPR_iCurr*BSPR_iCurr;
    BSER_cntCurrSqProc=0;
  state Time10msProc_stt
    entry:
    BSER_iCurrSqProcTmp=BSER_iCurrSqProcTmp+BSPR_iCurr*BSPR_iCurr;
    BSER_cntCurrSqProc=BSER_cntCurrSqProc+1;
    during:
    BSER_iCurrSqProcTmp=BSER_iCurrSqProcTmp+BSPR_iCurr*BSPR_iCurr;
    BSER_cntCurrSqProc=BSER_cntCurrSqProc+1;
  (default) -> (junction 67) : {i=0;}
  (junction 67) -> (junction 70) : [i<=9]
  (junction 70) -> (junction 71) : {BSER_iCurrSqProcTmp_A[i]=0;}
  (junction 71) -> (junction 67) : {i = i + 1;}
  (junction 67) -> (junction 68) : {Index_s=0;}
  (junction 68) -> (junction 78) : [Index_s<60]
  (junction 78) -> (junction 77) : {BSER_iCurrSqAvrgS_A[Index_s]=0;}
  (junction 77) -> (junction 68) : {Index_s = Index_s + 1;}
  (junction 68) -> Time10msStrt_stt1 : {i=0; Index_s=0;}
  Time10msStrt_stt1 -> Time10msProc_stt
  Time10msProc_stt -> Time100msProc_stt : [BSER_cntCurrSqProc>=9]
  (junction 43) -> Time10msProc_stt
  Time100msProc_stt -> (junction 43) : {i=i+1;}
  (junction 43) -> (junction 41) : [i>9]
  (junction 52) -> Time10msProc_stt : {Index_s=0;}
  (junction 55) -> Time10msProc_stt
  (junction 41) -> (junction 83) : {i=0;BSER_iCurrSqAvrgS=0;}
  (junction 36) -> (junction 83) : {i = i + 1;}
  (junction 83) -> (junction 38)
  (junction 39) -> (junction 36) : {BSER_iCurrSqAvrgS=BSER_iCurrSqAvrgS... +BSER_iCurrSqProcTmp_A[i];}
  (junction 55) -> (junction 52) : [Index_s>=BSER_tiCurrCalcPer_C]
  (junction 38) -> (junction 55) : {i=0; BSER_iCurrSqAvrgS_A[Index_s]=BSER_iCurrSqAvrgS/10; Index_s=Index_s+1;}
  (junction 38) -> (junction 39) : [i<=9]
  data: BSER_iCurrSqProcTmp_A local single; BSER_iCurrSqAvrgS local single; BSER_iCurrSqAvrgS_A output single; Index_s output uint8; BSPR_iCurr input; BSER_tiCurrCalcPer_C input; BSER_iCurrSqProcTmp local single; i output uint8; BSER_cntCurrSqProc local uint8

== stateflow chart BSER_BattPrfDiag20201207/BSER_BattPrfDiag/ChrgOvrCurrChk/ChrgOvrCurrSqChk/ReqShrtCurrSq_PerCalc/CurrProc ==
  state Time10msStrt_stt1
    entry:
    BSER_iCurrSqProcTmp=BSPR_iCurr*BSPR_iCurr;
    BSER_cntCurrSqProc=0;
  state Time100msProc_stt
    entry:
    BSER_iCurrSqProcTmp_A[i]=BSER_iCurrSqProcTmp/10;
    BSER_iCurrSqProcTmp=BSPR_iCurr*BSPR_iCurr;
    BSER_cntCurrSqProc=0;
  state Time10msProc_stt
    entry:
    BSER_iCurrSqProcTmp=BSER_iCurrSqProcTmp+BSPR_iCurr*BSPR_iCurr;
    BSER_cntCurrSqProc=BSER_cntCurrSqProc+1;
    during:
    BSER_iCurrSqProcTmp=BSER_iCurrSqProcTmp+BSPR_iCurr*BSPR_iCurr;
    BSER_cntCurrSqProc=BSER_cntCurrSqProc+1;
  (default) -> (junction 67) : {i=0;}
  (junction 67) -> (junction 70) : [i<=9]
  (junction 70) -> (junction 71) : {BSER_iCurrSqProcTmp_A[i]=0;}
  (junction 71) -> (junction 67) : {i = i + 1;}
  (junction 67) -> (junction 68) : {Index_s=0;}
  (junction 68) -> (junction 78) : [Index_s<60]
  (junction 78) -> (junction 77) : {BSER_iCurrSqAvrgS_A[Index_s]=0;}
  (junction 77) -> (junction 68) : {Index_s = Index_s + 1;}
  (junction 68) -> Time10msStrt_stt1 : {i=0; Index_s=0;}
  Time10msStrt_stt1 -> Time10msProc_stt
  Time10msProc_stt -> Time100msProc_stt : [BSER_cntCurrSqProc>=9]
  (junction 43) -> Time10msProc_stt
  Time100msProc_stt -> (junction 43) : {i=i+1;}
  (junction 43) -> (junction 41) : [i>9]
  (junction 52) -> Time10msProc_stt : {Index_s=0;}
  (junction 55) -> Time10msProc_stt
  (junction 41) -> (junction 83) : {i=0;BSER_iCurrSqAvrgS=0;}
  (junction 36) -> (junction 83) : {i = i + 1;}
  (junction 83) -> (junction 38)
  (junction 39) -> (junction 36) : {BSER_iCurrSqAvrgS=BSER_iCurrSqAvrgS... +BSER_iCurrSqProcTmp_A[i];}
  (junction 55) -> (junction 52) : [Index_s>=BSER_tiCurrCalcPer_C]
  (junction 38) -> (junction 55) : {i=0; BSER_iCurrSqAvrgS_A[Index_s]=BSER_iCurrSqAvrgS/10; Index_s=Index_s+1;}
  (junction 38) -> (junction 39) : [i<=9]
  data: BSER_iCurrSqProcTmp_A local single; BSER_iCurrSqAvrgS local single; BSER_iCurrSqAvrgS_A output single; Index_s output uint8; BSPR_iCurr input; BSER_tiCurrCalcPer_C input; BSER_iCurrSqProcTmp local single; i output uint8; BSER_cntCurrSqProc local uint8

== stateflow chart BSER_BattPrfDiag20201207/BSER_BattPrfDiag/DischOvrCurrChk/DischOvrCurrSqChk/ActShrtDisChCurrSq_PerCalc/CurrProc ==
  state Time10msStrt_stt1
    entry:
    BSER_iCurrSqProcTmp=BSPR_iCurr*BSPR_iCurr;
    BSER_cntCurrSqProc=0;
  state Time100msProc_stt
    entry:
    BSER_iCurrSqProcTmp_A[i]=BSER_iCurrSqProcTmp/10;
    BSER_iCurrSqProcTmp=BSPR_iCurr*BSPR_iCurr;
    BSER_cntCurrSqProc=0;
  state Time10msProc_stt
    entry:
    BSER_iCurrSqProcTmp=BSER_iCurrSqProcTmp+BSPR_iCurr*BSPR_iCurr;
    BSER_cntCurrSqProc=BSER_cntCurrSqProc+1;
    during:
    BSER_iCurrSqProcTmp=BSER_iCurrSqProcTmp+BSPR_iCurr*BSPR_iCurr;
    BSER_cntCurrSqProc=BSER_cntCurrSqProc+1;
  (default) -> (junction 67) : {i=0;}
  (junction 67) -> (junction 70) : [i<=9]
  (junction 70) -> (junction 71) : {BSER_iCurrSqProcTmp_A[i]=0;}
  (junction 71) -> (junction 67) : {i = i + 1;}
  (junction 67) -> (junction 68) : {Index_s=0;}
  (junction 68) -> (junction 78) : [Index_s<60]
  (junction 78) -> (junction 77) : {BSER_iCurrSqAvrgS_A[Index_s]=0;}
  (junction 77) -> (junction 68) : {Index_s = Index_s + 1;}
  (junction 68) -> Time10msStrt_stt1 : {i=0; Index_s=0;}
  Time10msStrt_stt1 -> Time10msProc_stt
  Time10msProc_stt -> Time100msProc_stt : [BSER_cntCurrSqProc>=9]
  (junction 43) -> Time10msProc_stt
  Time100msProc_stt -> (junction 43) : {i=i+1;}
  (junction 43) -> (junction 41) : [i>9]
  (junction 52) -> Time10msProc_stt : {Index_s=0;}
  (junction 55) -> Time10msProc_stt
  (junction 41) -> (junction 83) : {i=0;BSER_iCurrSqAvrgS=0;}
  (junction 36) -> (junction 83) : {i = i + 1;}
  (junction 83) -> (junction 38)
  (junction 39) -> (junction 36) : {BSER_iCurrSqAvrgS=BSER_iCurrSqAvrgS... +BSER_iCurrSqProcTmp_A[i];}
  (junction 55) -> (junction 52) : [Index_s>=BSER_tiCurrCalcPer_C]
  (junction 38) -> (junction 55) : {i=0; BSER_iCurrSqAvrgS_A[Index_s]=BSER_iCurrSqAvrgS/10; Index_s=Index_s+1;}
  (junction 38) -> (junction 39) : [i<=9]
  data: BSER_iCurrSqProcTmp_A local single; BSER_iCurrSqAvrgS local single; BSER_iCurrSqAvrgS_A output single; Index_s output uint8; BSPR_iCurr input; BSER_tiCurrCalcPer_C input; BSER_iCurrSqProcTmp local single; i output uint8; BSER_cntCurrSqProc local uint8

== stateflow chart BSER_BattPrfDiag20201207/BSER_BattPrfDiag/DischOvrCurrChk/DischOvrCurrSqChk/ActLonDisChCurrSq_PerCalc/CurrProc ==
  state Time10msStrt_stt1
    entry:
    BSER_iCurrSqProcTmp=BSPR_iCurr*BSPR_iCurr;
    BSER_cntCurrSqProc=0;
  state Time100msProc_stt
    entry:
    BSER_iCurrSqProcTmp_A[i]=BSER_iCurrSqProcTmp/10;
    BSER_iCurrSqProcTmp=BSPR_iCurr*BSPR_iCurr;
    BSER_cntCurrSqProc=0;
  state Time10msProc_stt
    entry:
    BSER_iCurrSqProcTmp=BSER_iCurrSqProcTmp+BSPR_iCurr*BSPR_iCurr;
    BSER_cntCurrSqProc=BSER_cntCurrSqProc+1;
    during:
    BSER_iCurrSqProcTmp=BSER_iCurrSqProcTmp+BSPR_iCurr*BSPR_iCurr;
    BSER_cntCurrSqProc=BSER_cntCurrSqProc+1;
  (default) -> (junction 67) : {i=0;}
  (junction 67) -> (junction 70) : [i<=9]
  (junction 70) -> (junction 71) : {BSER_iCurrSqProcTmp_A[i]=0;}
  (junction 71) -> (junction 67) : {i = i + 1;}
  (junction 67) -> (junction 68) : {Index_s=0;}
  (junction 68) -> (junction 78) : [Index_s<60]
  (junction 78) -> (junction 77) : {BSER_iCurrSqAvrgS_A[Index_s]=0;}
  (junction 77) -> (junction 68) : {Index_s = Index_s + 1;}
  (junction 68) -> Time10msStrt_stt1 : {i=0; Index_s=0;}
  Time10msStrt_stt1 -> Time10msProc_stt
  Time10msProc_stt -> Time100msProc_stt : [BSER_cntCurrSqProc>=9]
  (junction 43) -> Time10msProc_stt
  Time100msProc_stt -> (junction 43) : {i=i+1;}
  (junction 43) -> (junction 41) : [i>9]
  (junction 52) -> Time10msProc_stt : {Index_s=0;}
  (junction 55) -> Time10msProc_stt
  (junction 41) -> (junction 83) : {i=0;BSER_iCurrSqAvrgS=0;}
  (junction 36) -> (junction 83) : {i = i + 1;}
  (junction 83) -> (junction 38)
  (junction 39) -> (junction 36) : {BSER_iCurrSqAvrgS=BSER_iCurrSqAvrgS... +BSER_iCurrSqProcTmp_A[i];}
  (junction 55) -> (junction 52) : [Index_s>=BSER_tiCurrCalcPer_C]
  (junction 38) -> (junction 55) : {i=0; BSER_iCurrSqAvrgS_A[Index_s]=BSER_iCurrSqAvrgS/10; Index_s=Index_s+1;}
  (junction 38) -> (junction 39) : [i<=9]
  data: BSER_iCurrSqProcTmp_A local single; BSER_iCurrSqAvrgS local single; BSER_iCurrSqAvrgS_A output single; Index_s output uint8; BSPR_iCurr input; BSER_tiCurrCalcPer_C input; BSER_iCurrSqProcTmp local single; i output uint8; BSER_cntCurrSqProc local uint8

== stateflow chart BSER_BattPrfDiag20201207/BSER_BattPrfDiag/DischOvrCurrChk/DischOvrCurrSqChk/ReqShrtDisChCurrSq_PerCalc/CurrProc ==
  state Time10msStrt_stt1
    entry:
    BSER_iCurrSqProcTmp=BSPR_iCurr*BSPR_iCurr;
    BSER_cntCurrSqProc=0;
  state Time100msProc_stt
    entry:
    BSER_iCurrSqProcTmp_A[i]=BSER_iCurrSqProcTmp/10;
    BSER_iCurrSqProcTmp=BSPR_iCurr*BSPR_iCurr;
    BSER_cntCurrSqProc=0;
  state Time10msProc_stt
    entry:
    BSER_iCurrSqProcTmp=BSER_iCurrSqProcTmp+BSPR_iCurr*BSPR_iCurr;
    BSER_cntCurrSqProc=BSER_cntCurrSqProc+1;
    during:
    BSER_iCurrSqProcTmp=BSER_iCurrSqProcTmp+BSPR_iCurr*BSPR_iCurr;
    BSER_cntCurrSqProc=BSER_cntCurrSqProc+1;
  (default) -> (junction 67) : {i=0;}
  (junction 67) -> (junction 70) : [i<=9]
  (junction 70) -> (junction 71) : {BSER_iCurrSqProcTmp_A[i]=0;}
  (junction 71) -> (junction 67) : {i = i + 1;}
  (junction 67) -> (junction 68) : {Index_s=0;}
  (junction 68) -> (junction 78) : [Index_s<60]
  (junction 78) -> (junction 77) : {BSER_iCurrSqAvrgS_A[Index_s]=0;}
  (junction 77) -> (junction 68) : {Index_s = Index_s + 1;}
  (junction 68) -> Time10msStrt_stt1 : {i=0; Index_s=0;}
  Time10msStrt_stt1 -> Time10msProc_stt
  Time10msProc_stt -> Time100msProc_stt : [BSER_cntCurrSqProc>=9]
  (junction 43) -> Time10msProc_stt
  Time100msProc_stt -> (junction 43) : {i=i+1;}
  (junction 43) -> (junction 41) : [i>9]
  (junction 52) -> Time10msProc_stt : {Index_s=0;}
  (junction 55) -> Time10msProc_stt
  (junction 41) -> (junction 83) : {i=0;BSER_iCurrSqAvrgS=0;}
  (junction 36) -> (junction 83) : {i = i + 1;}
  (junction 83) -> (junction 38)
  (junction 39) -> (junction 36) : {BSER_iCurrSqAvrgS=BSER_iCurrSqAvrgS... +BSER_iCurrSqProcTmp_A[i];}
  (junction 55) -> (junction 52) : [Index_s>=BSER_tiCurrCalcPer_C]
  (junction 38) -> (junction 55) : {i=0; BSER_iCurrSqAvrgS_A[Index_s]=BSER_iCurrSqAvrgS/10; Index_s=Index_s+1;}
  (junction 38) -> (junction 39) : [i<=9]
  data: BSER_iCurrSqProcTmp_A local single; BSER_iCurrSqAvrgS local single; BSER_iCurrSqAvrgS_A output single; Index_s output uint8; BSPR_iCurr input; BSER_tiCurrCalcPer_C input; BSER_iCurrSqProcTmp local single; i output uint8; BSER_cntCurrSqProc local uint8

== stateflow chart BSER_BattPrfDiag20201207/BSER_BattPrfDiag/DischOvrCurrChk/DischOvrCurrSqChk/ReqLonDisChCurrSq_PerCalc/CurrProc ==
  state Time10msStrt_stt1
    entry:
    BSER_iCurrSqProcTmp=BSPR_iCurr*BSPR_iCurr;
    BSER_cntCurrSqProc=0;
  state Time100msProc_stt
    entry:
    BSER_iCurrSqProcTmp_A[i]=BSER_iCurrSqProcTmp/10;
    BSER_iCurrSqProcTmp=BSPR_iCurr*BSPR_iCurr;
    BSER_cntCurrSqProc=0;
  state Time10msProc_stt
    entry:
    BSER_iCurrSqProcTmp=BSER_iCurrSqProcTmp+BSPR_iCurr*BSPR_iCurr;
    BSER_cntCurrSqProc=BSER_cntCurrSqProc+1;
    during:
    BSER_iCurrSqProcTmp=BSER_iCurrSqProcTmp+BSPR_iCurr*BSPR_iCurr;
    BSER_cntCurrSqProc=BSER_cntCurrSqProc+1;
  (default) -> (junction 67) : {i=0;}
  (junction 67) -> (junction 70) : [i<=9]
  (junction 70) -> (junction 71) : {BSER_iCurrSqProcTmp_A[i]=0;}
  (junction 71) -> (junction 67) : {i = i + 1;}
  (junction 67) -> (junction 68) : {Index_s=0;}
  (junction 68) -> (junction 78) : [Index_s<60]
  (junction 78) -> (junction 77) : {BSER_iCurrSqAvrgS_A[Index_s]=0;}
  (junction 77) -> (junction 68) : {Index_s = Index_s + 1;}
  (junction 68) -> Time10msStrt_stt1 : {i=0; Index_s=0;}
  Time10msStrt_stt1 -> Time10msProc_stt
  Time10msProc_stt -> Time100msProc_stt : [BSER_cntCurrSqProc>=9]
  (junction 43) -> Time10msProc_stt
  Time100msProc_stt -> (junction 43) : {i=i+1;}
  (junction 43) -> (junction 41) : [i>9]
  (junction 52) -> Time10msProc_stt : {Index_s=0;}
  (junction 55) -> Time10msProc_stt
  (junction 41) -> (junction 83) : {i=0;BSER_iCurrSqAvrgS=0;}
  (junction 36) -> (junction 83) : {i = i + 1;}
  (junction 83) -> (junction 38)
  (junction 39) -> (junction 36) : {BSER_iCurrSqAvrgS=BSER_iCurrSqAvrgS... +BSER_iCurrSqProcTmp_A[i];}
  (junction 55) -> (junction 52) : [Index_s>=BSER_tiCurrCalcPer_C]
  (junction 38) -> (junction 55) : {i=0; BSER_iCurrSqAvrgS_A[Index_s]=BSER_iCurrSqAvrgS/10; Index_s=Index_s+1;}
  (junction 38) -> (junction 39) : [i<=9]
  data: BSER_iCurrSqProcTmp_A local single; BSER_iCurrSqAvrgS local single; BSER_iCurrSqAvrgS_A output single; Index_s output uint8; BSPR_iCurr input; BSER_tiCurrCalcPer_C input; BSER_iCurrSqProcTmp local single; i output uint8; BSER_cntCurrSqProc local uint8

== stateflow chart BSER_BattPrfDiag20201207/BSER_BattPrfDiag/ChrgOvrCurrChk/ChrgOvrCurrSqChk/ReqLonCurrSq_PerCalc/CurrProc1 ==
  state Time10msStrt_stt1
    entry:
    BSER_iCurrSqProcTmp=BSPR_iCurr*BSPR_iCurr;
    BSER_cntCurrSqProc=0;
  state Time100msProc_stt
    entry:
    BSER_iCurrSqProcTmp_A[i]=BSER_iCurrSqProcTmp/10;
    BSER_iCurrSqProcTmp=BSPR_iCurr*BSPR_iCurr;
    BSER_cntCurrSqProc=0;
  state Time10msProc_stt
    entry:
    BSER_iCurrSqProcTmp=BSER_iCurrSqProcTmp+BSPR_iCurr*BSPR_iCurr;
    BSER_cntCurrSqProc=BSER_cntCurrSqProc+1;
    during:
    BSER_iCurrSqProcTmp=BSER_iCurrSqProcTmp+BSPR_iCurr*BSPR_iCurr;
    BSER_cntCurrSqProc=BSER_cntCurrSqProc+1;
  (default) -> (junction 67) : {i=0;}
  (junction 67) -> (junction 70) : [i<=9]
  (junction 70) -> (junction 71) : {BSER_iCurrSqProcTmp_A[i]=0;}
  (junction 71) -> (junction 67) : {i = i + 1;}
  (junction 67) -> (junction 68) : {Index_s=0;}
  (junction 68) -> (junction 78) : [Index_s<60]
  (junction 78) -> (junction 77) : {BSER_iCurrSqAvrgS_A[Index_s]=0;}
  (junction 77) -> (junction 68) : {Index_s = Index_s + 1;}
  (junction 68) -> Time10msStrt_stt1 : {i=0; Index_s=0;}
  Time10msStrt_stt1 -> Time10msProc_stt
  Time10msProc_stt -> Time100msProc_stt : [BSER_cntCurrSqProc>=9]
  (junction 43) -> Time10msProc_stt
  Time100msProc_stt -> (junction 43) : {i=i+1;}
  (junction 43) -> (junction 41) : [i>9]
  (junction 52) -> Time10msProc_stt : {Index_s=0;}
  (junction 55) -> Time10msProc_stt
  (junction 41) -> (junction 83) : {i=0;BSER_iCurrSqAvrgS=0;}
  (junction 36) -> (junction 83) : {i = i + 1;}
  (junction 83) -> (junction 38)
  (junction 39) -> (junction 36) : {BSER_iCurrSqAvrgS=BSER_iCurrSqAvrgS... +BSER_iCurrSqProcTmp_A[i];}
  (junction 55) -> (junction 52) : [Index_s>=BSER_tiCurrCalcPer_C]
  (junction 38) -> (junction 55) : {i=0; BSER_iCurrSqAvrgS_A[Index_s]=BSER_iCurrSqAvrgS/10; Index_s=Index_s+1;}
  (junction 38) -> (junction 39) : [i<=9]
  data: BSER_iCurrSqProcTmp_A local single; BSER_iCurrSqAvrgS local single; BSER_iCurrSqAvrgS_A output single; Index_s output uint8; BSPR_iCurr input; BSER_tiCurrCalcPer_C input; BSER_iCurrSqProcTmp local single; i output uint8; BSER_cntCurrSqProc local uint8
